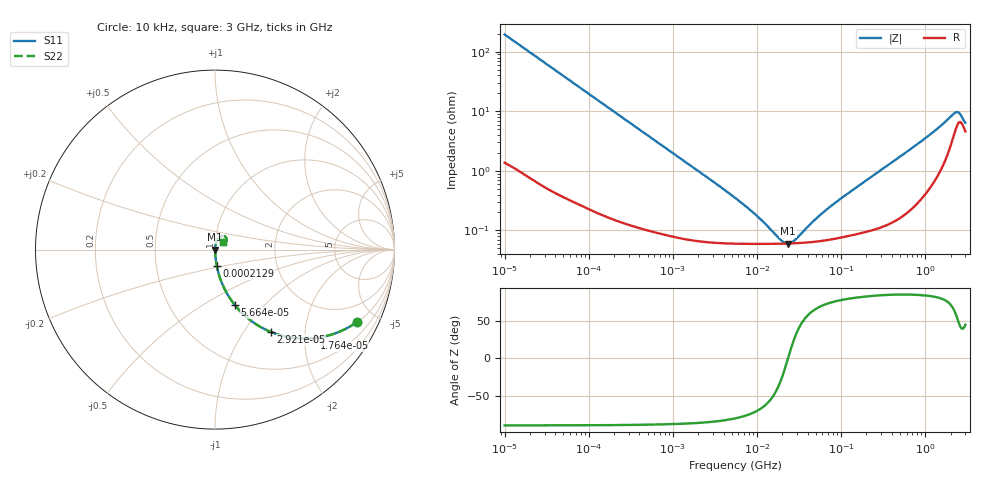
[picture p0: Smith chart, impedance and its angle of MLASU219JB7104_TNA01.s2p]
! MLASU219JB7104_TNA01  S-PARAMETER MODEL  ( Standard Model )
! Model Generated by TAIYO YUDEN Corporation (http://www.ty-top.com)
! Version 1.0
! TAIYO YUDEN Control No. 220601
! Copyright(c) 2011 TAIYO YUDEN CO.,LTD. All Rights Reserved.
! Product Description (link to TY-COMPAS)
! https://ds.yuden.co.jp/TYCOMPAS/or/detail?pn=MLASU219JB7104KTNA01&u=M
! Products Name : Multilayer Ceramic Capacitors
! Characteristics :
!  Capacitance : 0.1 [uF] , Rated Voltage : 50 [V] , TCC : X7R
!  Case Size : 2.0 x 1.25 / 0.079 x 0.049 [mm/inch] , Thickness : 0.85 / 0.033 [mm/inch]
!  (Conditions: Temperature = 25 [degC] , DC Bias Voltage = 0 [V])
! External Node Assignments :
!  1  o---| |---o  2
! GND o---------o GND
! Frequency Range : 10kHz  -  3GHz  [ 401 STEP ]
# MHZ S RI R 50
! Freq[MHz].  S11 Real  S11 Imag  S21 Real  S21 Imag  S12 Real  S12 Imag  S22 Real  S22 Imag
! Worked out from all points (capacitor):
!   401 points, 10 kHz to 3 GHz, reference 50 ohm
!   read as one part in series: C = 81.5 nF near 10.65 kHz
!   lowest |Z| = 60.3 mohm at 23.36 MHz (marker M1)
!   series resonance near 23.4 MHz, so ESL is about 570 pH
!   S11 on the Smith chart (normalised r, x): 10 kHz: 1.03, -3.90; 17.64 kHz: 1.02, -2.22; 29.21 kHz: 1.01, -1.34; 56.64 kHz: 1.01, -0.69; 212.9 kHz: 1.00, -0.19; 3 GHz: 1.09, +0.09
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0.01  0.7902 -0.4037  0.2098 0.4037  0.2098 0.4037  0.7902 -0.4037
0.01247  0.709 -0.4506  0.291 0.4506  0.291 0.4506  0.709 -0.4506
0.017639  0.5512 -0.4936  0.4488 0.4936  0.4488 0.4936  0.5512 -0.4936
0.022699  0.4273 -0.4908  0.5727 0.4908  0.5727 0.4908  0.4273 -0.4908
0.029212  0.312 -0.4593  0.688 0.4593  0.688 0.4593  0.312 -0.4593
0.040039  0.1959 -0.3926  0.8041 0.3926  0.8041 0.3926  0.1959 -0.3926
0.056638  0.1099 -0.308  0.8901 0.308  0.8901 0.308  0.1099 -0.308
0.082683  0.0559 -0.2244  0.9441 0.2244  0.9441 0.2244  0.0559 -0.2244
0.212913  0.01 -0.092  0.99 0.092  0.99 0.092  0.01 -0.092
0.683653  0.00174 -0.0291  0.9983 0.0291  0.9983 0.0291  0.00174 -0.0291
5.477226  0.000611 -0.00348  0.9994 0.00348  0.9994 0.00348  0.000611 -0.00348
10.29003  0.000596 -0.00158  0.9994 0.00158  0.9994 0.00158  0.000596 -0.00158
19.33182  0.000598 -0.00033  0.9994 0.00033  0.9994 0.00033  0.000598 -0.00033
23.35767  0.000602 -3.05e-06  0.9994 3.05e-06  0.9994 3.05e-06  0.000602 -3.05e-06
28.22191  0.000609 0.000324  0.9994 -0.000324  0.9994 -0.000324  0.000609 0.000324
45.28751  0.000639 0.00121  0.9994 -0.00121  0.9994 -0.00121  0.000639 0.00121
90.61918  0.000747 0.00302  0.9993 -0.00302  0.9993 -0.00302  0.000747 0.00302
374.4521  0.00144 0.0128  0.9986 -0.0128  0.9986 -0.0128  0.00144 0.0128
1128.871  0.00662 0.0395  0.9934 -0.0395  0.9934 -0.0395  0.00662 0.0395
2188.735  0.0443 0.0759  0.9557 -0.0759  0.9557 -0.0759  0.0443 0.0759
2482.93  0.0642 0.0629  0.9358 -0.0629  0.9358 -0.0629  0.0642 0.0629
3000  0.0457 0.0412  0.9543 -0.0412  0.9543 -0.0412  0.0457 0.0412
